TYPE E_StateSeparatingAuto :
(
	eSeparatingAuto_Init	:= 0,
	eSeparatingAuto_Start,
	eSeparatingAuto_CloseClamp,
	eSeparatingAuto_OpenBarrier,
	eSeparatingAuto_CloseBarrier,
	eSeparatingAuto_OpenClamp
);
END_TYPE
